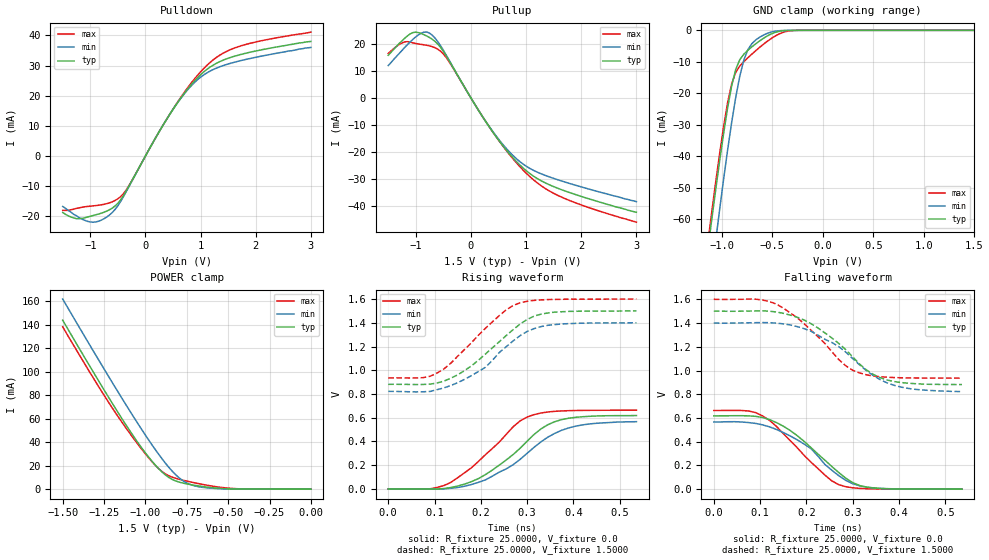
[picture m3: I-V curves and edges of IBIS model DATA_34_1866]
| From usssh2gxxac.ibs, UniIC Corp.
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|   Model DATA_34_1866
[Model]  DATA_34_1866
Model_type I/O
Polarity   Non-Inverting
Enable   Active-High
Vinl =   0.61500000V
Vinh =   0.88500000V
Vmeas =   0.750000000V
Rref =   25.00000000
Vref =   0.75000000V
C_comp   1.6160pF   1.5990pF   1.6430pF
[Temperature Range]   25.0000   95.0000   0.0
[Voltage Range]   1.5000V   1.4000V   1.6000V
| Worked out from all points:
|   slope of the pulldown table from 0 to 0.225 V, typ, clamps not added: 30.8 ohm
|   slope of the pullup table from 0 to 0.225 V, typ, clamps not added: 30.4 ohm
|   GND clamp passes 1 mA (typ) near -0.50 V on its own axis
|   POWER clamp passes 1 mA (typ) near -0.58 V on its own axis
|   rising waveform, R_fixture 25.0000, V_fixture 0.0: 20-80 % time 115ps typ, 125ps min, 108ps max; typ from 0 V to 0.618 V
|   rising waveform, R_fixture 25.0000, V_fixture 1.5000: 20-80 % time 113ps typ, 111ps min, 104ps max; typ from 0.881 V to 1.5 V
|   falling waveform, R_fixture 25.0000, V_fixture 0.0: 20-80 % time 110ps typ, 107ps min, 101ps max; typ from 0.618 V to 0 V
|   falling waveform, R_fixture 25.0000, V_fixture 1.5000: 20-80 % time 112ps typ, 122ps min, 105ps max; typ from 1.5 V to 0.882 V
[Pulldown]
|Voltage   I(typ)   I(min)   I(max)
-1.5V     -18.7mA    -16.7mA    -18mA
-1.25V    -20.76mA   -19.8mA    -17.33mA
-1V       -19.96mA   -21.85mA   -16.61mA
-800mV    -18.94mA   -21.24mA   -16.16mA
-600mV    -17.23mA   -18.69mA   -15.15mA
-350mV    -11.62mA   -11.84mA   -11.29mA
200mV     6.523mA    6.58mA     6.518mA
550mV     16.83mA    16.81mA    16.97mA
850mV     24.09mA    23.66mA    24.66mA
1.15V     29.22mA    27.95mA    30.67mA
1.7V      33.54mA    31.52mA    36.35mA
3V        38mA       36mA       41.1mA
[Pullup]
|Voltage   I(typ)   I(min)   I(max)
-1.5V     15.8mA     12mA       16.5mA
-1.25V    21.14mA    17.6mA     20.39mA
-1.05V    24.23mA    21.76mA    20.4mA
-900mV    23.84mA    24.02mA    19.83mA
-750mV    22.38mA    24mA       19.29mA
-600mV    19.94mA    20.83mA    18.05mA
-450mV    15.66mA    15.92mA    15.03mA
300mV     -9.744mA   -9.622mA   -9.709mA
850mV     -24.07mA   -22.95mA   -24.6mA
1.2V      -29.82mA   -27.44mA   -31.4mA
1.55V     -33.24mA   -30.13mA   -35.83mA
3V        -42.3mA    -38.4mA    -46mA
[GND_clamp]
|Voltage   I(typ)   I(min)   I(max)
-1.5V     -169mA     -189.1mA   -163.8mA
-1.14V    -70.71mA   -88.3mA    -68.32mA
-1.1V     -60.74mA   -77.66mA   -58.33mA
-1.06V    -51.03mA   -67.22mA   -48.61mA
-1.02V    -41.65mA   -57.06mA   -39.27mA
-940mV    -24.55mA   -37.9mA    -22.88mA
-860mV    -12.39mA   -21.26mA   -13.32mA
-780mV    -7.577mA   -9.433mA   -9.942mA
-740mV    -6.329mA   -6.125mA   -8.71mA
-620mV    -3.273mA   -2.113mA   -5.305mA
-300mV    -11.81uA   -4.878uA   -91.71uA
1.5V      4.577nA    23.6nA     33.33nA
[POWER_clamp]
|Voltage   I(typ)   I(min)   I(max)
-1.5V     143.7mA    161.7mA    138.1mA
-1.22V    77.56mA    95.29mA    73.32mA
-1.12V    55.19mA    72.34mA    52.54mA
-1.02V    34.59mA    50.23mA    33.56mA
-960mV    23.77mA    37.63mA    23.28mA
-900mV    14.66mA    25.9mA     15mA
-840mV    8.415mA    15.63mA    10.28mA
-780mV    5.408mA    7.848mA    7.861mA
-700mV    3.206mA    2.693mA    5.332mA
-600mV    1.29mA     794.5uA    2.681mA
-420mV    69.47uA    44.47uA    238.7uA
0V        4.577nA    6.249nA    39.08nA
[Ramp]
| variable   typ   min   max
dV/dt_r  0.3707/0.1151n   0.3398/0.1312n   0.3978/0.1081n
dV/dt_f  0.3712/0.1121n   0.3468/0.1264n   0.3986/0.1049n
R_load = 25.0000
[Rising Waveform]
R_fixture= 25.0000
V_fixture= 0.0
V_fixture_min= 0.0
V_fixture_max= 0.0
|time   V(typ)   V(min)   V(max)
0s        0V         0V         0V
90.91ps   -832.3uV   -33.66uV   979.3uV
135ps     11.16mV    4.781mV    54.16mV
180ps     61.22mV    37.02mV    178.8mV
210ps     120.4mV    75.74mV    288.6mV
285ps     343.1mV    249.4mV    573.3mV
315ps     458.9mV    350.4mV    625.9mV
360ps     566.8mV    468.6mV    653.7mV
405ps     603.3mV    528.8mV    660.6mV
536ps     617.9mV    566.4mV    663mV
[Rising Waveform]
R_fixture= 25.0000
V_fixture= 1.5000
V_fixture_min= 1.4000
V_fixture_max= 1.6000
|time   V(typ)   V(min)   V(max)
0s        881.4mV    822mV      935.7mV
75.76ps   880.1mV    818.6mV    937.7mV
105ps     891.6mV    835.6mV    975.2mV
150ps     961.6mV    895.1mV    1.118V
210ps     1.137V     1.025V     1.354V
255ps     1.293V     1.199V     1.51V
285ps     1.39V      1.292V     1.569V
315ps     1.456V     1.351V     1.589V
360ps     1.49V      1.385V     1.597V
536ps     1.5V       1.4V       1.6V
[Falling Waveform]
R_fixture= 25.0000
V_fixture= 0.0
V_fixture_min= 0.0
V_fixture_max= 0.0
|time   V(typ)   V(min)   V(max)
0s        617.9mV    566.4mV    662.9mV
75.76ps   617.7mV    560.9mV    658.6mV
105ps     604mV      542.3mV    618.1mV
150ps     531.4mV    477.7mV    468.6mV
210ps     350mV      341.6mV    227.3mV
240ps     243.9mV    208.2mV    118.6mV
270ps     140mV      113.3mV    37.86mV
300ps     55.27mV    45.68mV    11.55mV
330ps     17.27mV    17.46mV    3.695mV
536ps     0V         0V         0V
[Falling Waveform]
R_fixture= 25.0000
V_fixture= 1.5000
V_fixture_min= 1.4000
V_fixture_max= 1.6000
|time   V(typ)   V(min)   V(max)
0s        1.5V       1.4V       1.6V
90.91ps   1.502V     1.403V     1.601V
135ps     1.493V     1.399V     1.56V
180ps     1.449V     1.37V      1.445V
210ps     1.395V     1.331V     1.339V
285ps     1.176V     1.155V     1.04V
315ps     1.054V     1.047V     979.3mV
345ps     965.9mV    955.6mV    953.5mV
390ps     906.6mV    874.7mV    940.4mV
536ps     881.5mV    822.1mV    935.7mV
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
